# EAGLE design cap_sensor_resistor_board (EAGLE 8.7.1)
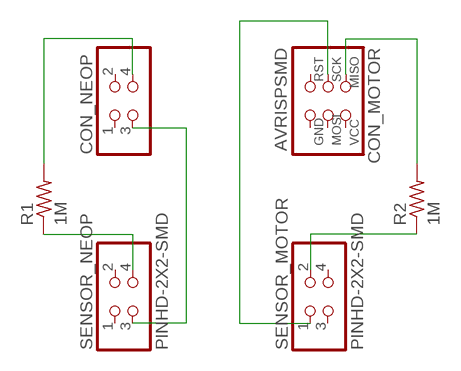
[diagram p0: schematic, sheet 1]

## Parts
CON_MOTOR  AVRISPSMD  [2X03SMD]
CON_NEOP  PINHD-2X2-SMD  [2X02SMD]
R1  1M  RES-US1206FAB  [R1206FAB]
R2  1M  RES-US1206FAB  [R1206FAB]
SENSOR_MOTOR  PINHD-2X2-SMD  [2X02SMD]
SENSOR_NEOP  PINHD-2X2-SMD  [2X02SMD]

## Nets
N$1: CON_MOTOR.1(MISO) R2.2
N$2: R2.1 SENSOR_MOTOR.2
N$3: CON_MOTOR.3(SCK) SENSOR_MOTOR.1
N$4: CON_NEOP.4 R1.2
N$5: R1.1 SENSOR_NEOP.4
N$6: CON_NEOP.3 SENSOR_NEOP.3
Unconnected: CON_MOTOR.2(VCC) CON_MOTOR.4(MOSI) CON_MOTOR.5(RST) CON_MOTOR.6(GND) CON_NEOP.1 CON_NEOP.2 SENSOR_MOTOR.3 SENSOR_MOTOR.4 SENSOR_NEOP.1 SENSOR_NEOP.2

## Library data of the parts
CON_MOTOR = fab:AVRISP
CON_NEOP SENSOR_MOTOR SENSOR_NEOP = fab:PINHD-2X2-SMD
R1 R2 = fab:RES-US: Resistor (US Symbol)

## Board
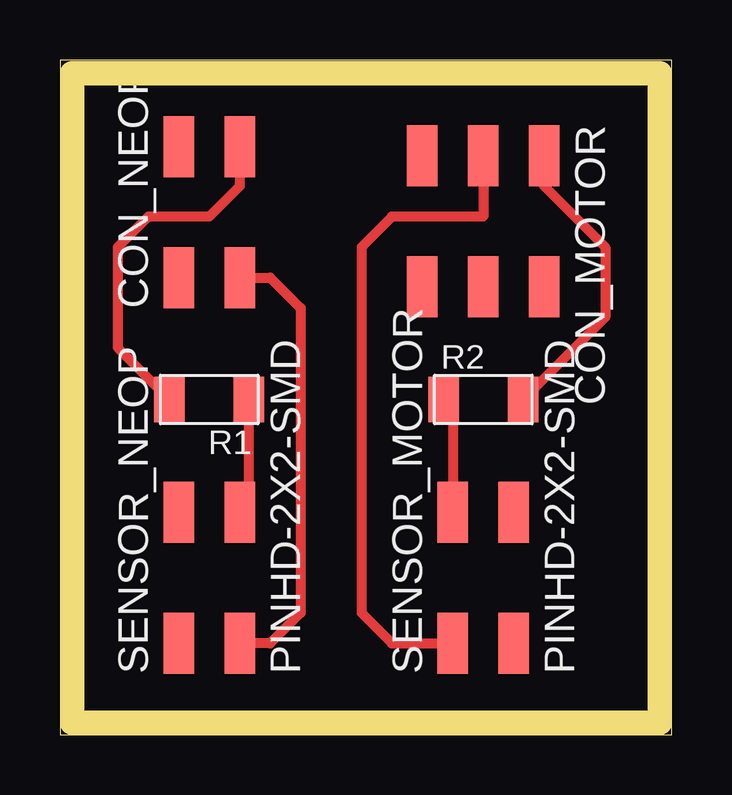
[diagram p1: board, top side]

Size 25.51 x 28.12 mm. Coordinates in mm from the lower left corner, seen from the top.
Outline: 0,0 25.51,0 25.51,28.12 0,28.12 0,0
Copper layers (1*16): Top 0.035mm / dielectric 1.5mm / Bottom 0.035mm
Design rules "default *": minimum track width 16mil, minimum drill 0.35mm, track to track 16mil, track to pad 16mil, pad to pad 16mil, via to via 16mil, smd to smd 16mil, copper to edge 40mil, drill to drill 16mil, minimum pad ring 10mil, minimum via ring 8mil, stop-mask expansion 4mil, vias tented up to drill 0mil, thermal gap 10mil
Milling: 4 lines

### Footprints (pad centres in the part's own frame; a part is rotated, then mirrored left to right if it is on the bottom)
2X03SMD = smd 2.54 x 1.27: 1 -2.54,2.54; 2 2.92,2.54; 3 -2.54,0; 4 2.92,0; 5 -2.54,-2.54; 6 2.92,-2.54
2X02SMD = smd 2.54 x 1.27: 1 -2.54,1.27; 2 2.92,1.27; 3 -2.54,-1.27; 4 2.92,-1.27
R1206FAB = smd 1.27 x 1.905: 1 -1.651,0; 2 1.651,0

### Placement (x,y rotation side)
CON_MOTOR  17.65,21.59 270 top
CON_NEOP  6.22,21.59 90 top
R1  6.22,13.97 180 top
R2  17.65,13.97 0 top
SENSOR_MOTOR  17.65,6.35 90 top
SENSOR_NEOP  6.22,6.35 90 top

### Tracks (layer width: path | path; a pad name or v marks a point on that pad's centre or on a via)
N$1
  Top 0.406: CON_MOTOR.1 20.19,22.86 22.73,20.32 22.73,17.4 R2.2
N$2
  Top 0.406: R2.1 16.38,13.59 SENSOR_MOTOR.2
N$3
  Top 0.406: CON_MOTOR.3 17.65,21.59 13.84,21.59 12.57,20.32 12.57,5.08 13.84,3.81 SENSOR_MOTOR.1
N$4
  Top 0.406: CON_NEOP.4 7.49,22.86 6.22,21.59 3.68,21.59 2.41,20.32 2.41,16.13 R1.2
N$5
  Top 0.406: R1.1 7.87,9.65 SENSOR_NEOP.4
N$6
  Top 0.406: CON_NEOP.3 8.76,19.05 10.03,17.78 10.03,5.08 8.76,3.81 SENSOR_NEOP.3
